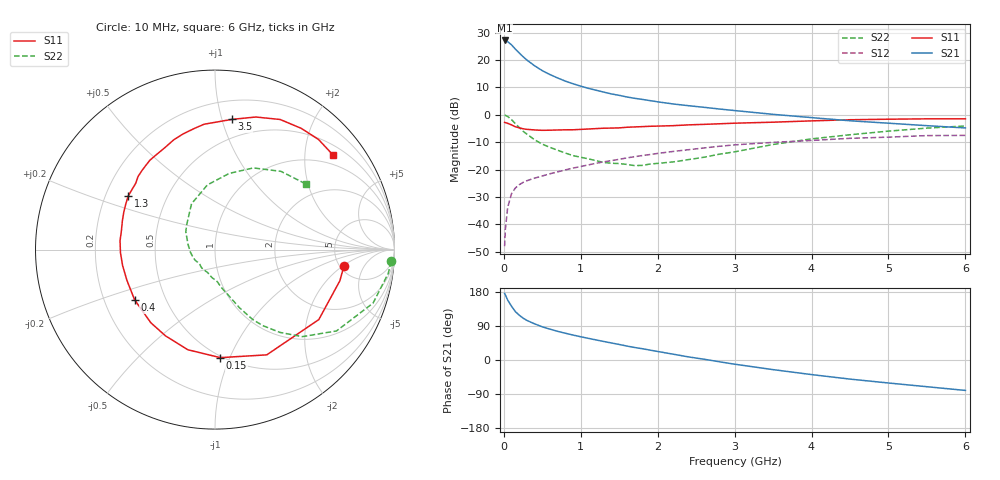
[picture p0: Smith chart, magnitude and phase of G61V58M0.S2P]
! SIEMENS Small Signal Semiconductors
! BFG193
! Si NPN RF Bipolar Junction Transistor in SOT223
! VCE = 1.5 V  IC = 8 mA
! Common Emitter S-Parameters:  August  1996
# GHz  S  MA  R  50
!  f  S11  S21  S12  S22
! GHz  MAG  ANG  MAG  ANG  MAG  ANG  MAG  ANG
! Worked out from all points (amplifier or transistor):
!   36 points, 10 MHz to 6 GHz, reference 50 ohm
!   highest |S21| = 27.1 dB at 10 MHz (marker M1)
!   |S21| within 3 dB of that: start of sweep to 144.7 MHz
!   unconditionally stable (mu >= 1): 909 MHz to 2.778 GHz
!   at 250 MHz: K = 0.47, MSG = 22.9 dB, |S12| = -24.7 dB
!   at 1.4 GHz: K = 1.08, MAG = 10.4 dB, |S12| = -16.7 dB
!   at 6 GHz: K = 0.94, MSG = 1.4 dB, |S12| = -7.5 dB
!   S11 on the Smith chart (normalised r, x): 10 MHz: 5.46, -2.06; 150 MHz: 0.49, -0.92; 400 MHz: 0.33, -0.26; 1.3 GHz: 0.30, +0.26; 3.5 GHz: 0.35, +1.08; 6 GHz: 0.74, +2.68
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0.01  0.7244 -7.1  22.67 175.5  0.004 89.7  0.9829 -3.8
0.02  0.7171 -14.0  22.62 171.7  0.0082 82.6  0.9745 -7.8
0.05  0.6975 -34.0  21.56 158.1  0.0204 73.7  0.9298 -18.7
0.1  0.6535 -63.8  18.84 141.9  0.0363 62.7  0.8147 -33.8
0.15  0.6027 -87.2  15.74 127.6  0.0461 53.6  0.687 -44.9
0.2  0.5781 -105.2  13.44 118.3  0.0529 49.6  0.5862 -51.9
0.25  0.5542 -119.8  11.46 110.5  0.0583 46.1  0.5008 -57.8
0.3  0.5421 -131.3  9.947 104.4  0.0626 44.7  0.4421 -61.7
0.4  0.5282 -148.0  7.823 95.4  0.0698 43.3  0.3497 -67.3
0.5  0.5198 -160.7  6.371 87.5  0.0763 43.0  0.2906 -71.3
0.6  0.5225 -170.4  5.406 81.4  0.0838 43.4  0.2538 -74.8
0.7  0.5271 -178.3  4.684 75.6  0.0907 43.5  0.2251 -78.8
0.9  0.532 168.5  3.673 65.8  0.1064 43.6  0.1797 -85.8
1.1  0.5494 157.7  3.031 57.1  0.1218 42.9  0.1566 -96.3
1.3  0.5683 148.3  2.585 48.8  0.1385 41.1  0.1345 -107.5
1.7  0.5992 132.9  1.995 33.0  0.1716 36.4  0.1179 -136.4
2.2  0.6321 116.5  1.573 15.4  0.2139 27.7  0.1377 -173.8
2.8  0.6838 100.0  1.273 -4.6  0.2658 15.9  0.1907 148.6
3.5  0.7316 82.6  1.017 -25.4  0.3135 -0.2  0.287 117.1
4.5  0.8107 63.4  0.776 -50.4  0.3715 -19.7  0.4315 79.5
5.5  0.8421 46.8  0.632 -70.5  0.4165 -43.1  0.5701 49.9
6  0.8431 38.5  0.574 -80.3  0.4197 -56.6  0.6242 35.9
